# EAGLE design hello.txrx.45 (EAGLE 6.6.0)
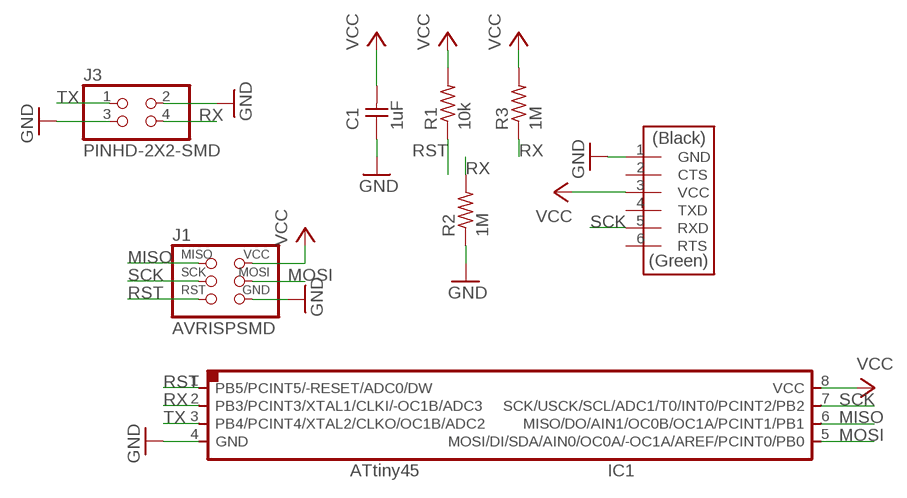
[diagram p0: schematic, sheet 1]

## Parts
C1  1uF  CAP-UNPOLARIZEDFAB  [C1206FAB]
IC1  ATTINY45SI  [SOIC8]
J1  AVRISPSMD  [2X03SMD]
J2  FTDI-SMD-HEADER  [1X06SMD]
J3  PINHD-2X2-SMD  [2X02SMD]
R1  10k  RES-US1206FAB  [R1206FAB]
R2  1M  RES-US1206FAB  [R1206FAB]
R3  1M  RES-US1206FAB  [R1206FAB]

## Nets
GND: C1.1 IC1.4(GND) J1.6(GND) J2.1(GND) J3.2 J3.3 R2.1
MISO: IC1.6(MISO/DO/AIN1/OC0B/OC1A/PCINT1/PB1) J1.1(MISO)
MOSI: IC1.5(MOSI/DI/SDA/AIN0/OC0A/-OC1A/AREF/PCINT0/PB0) J1.4(MOSI)
RST: IC1.1(PB5/PCINT5/-RESET/ADC0/DW) J1.5(RST) R1.1
RX: IC1.2(PB3/PCINT3/XTAL1/CLKI/-OC1B/ADC3) J3.4 R2.2 R3.1
SCK: IC1.7(SCK/USCK/SCL/ADC1/T0/INT0/PCINT2/PB2) J1.3(SCK) J2.5(RXD)
TX: IC1.3(PB4/PCINT4/XTAL2/CLKO/OC1B/ADC2) J3.1
VCC: C1.2 IC1.8(VCC) J1.2(VCC) J2.3(VCC) R1.2 R3.2
Unconnected: J2.2(CTS) J2.4(TXD) J2.6(RTS)

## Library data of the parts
C1 = fab:CAP-UNPOLARIZED
IC1 = fab:ATTINY45
J1 = fab:AVRISP
J2 = fab:FTDI-SMD-HEADER
J3 = fab:PINHD-2X2-SMD
R1-R3 = fab:RES-US: Resistor (US Symbol)

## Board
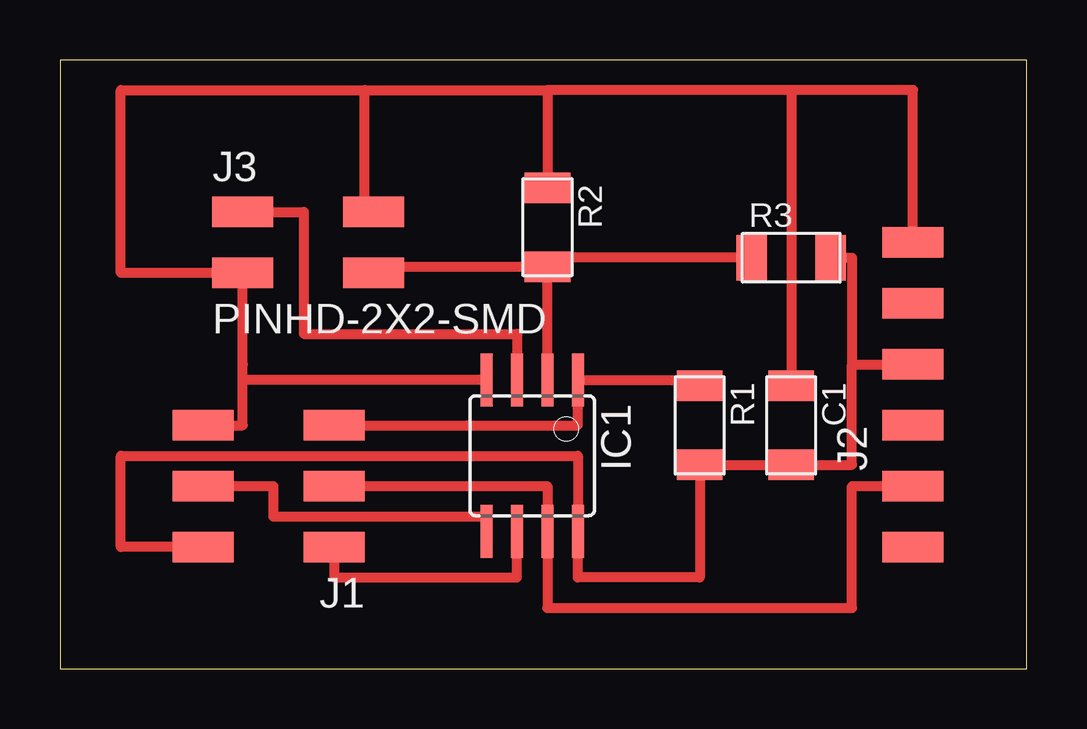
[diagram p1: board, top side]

Size 40.31 x 25.39 mm. Coordinates in mm from the lower left corner, seen from the top.
Outline: 0,0 40.31,0 40.31,25.39 0,25.39 0,0
Copper layers (1*16): Top 0.035mm / dielectric 1.5mm / Bottom 0.035mm
Design rules "fabmodule": minimum track width 10mil, minimum drill 0.4mm, track to track 0.42mm, track to pad 0.42mm, pad to pad 0.42mm, via to via 0.42mm, smd to smd 0.42mm, copper to edge 40mil, drill to drill 0.8mm, minimum pad ring 10mil, minimum via ring 8mil, stop-mask expansion 4mil, vias tented up to drill 0mil, thermal gap 10mil

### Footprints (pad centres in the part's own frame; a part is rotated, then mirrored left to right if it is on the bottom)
C1206FAB = smd 1.27 x 1.905: 1 -1.651,0; 2 1.651,0
SOIC8 = smd 0.5 x 2.2: 1 -1.905,-3.154; 2 -0.645,-3.154; 3 0.625,-3.154; 4 1.895,-3.154; 5 1.905,3.154; 6 0.635,3.154; 7 -0.635,3.154; 8 -1.905,3.154
2X03SMD = smd 2.54 x 1.27: 1 -2.54,2.54; 2 2.92,2.54; 3 -2.54,0; 4 2.92,0; 5 -2.54,-2.54; 6 2.92,-2.54
1X06SMD = smd 2.54 x 1.27: 1 0,6.35; 2 0,3.81; 3 0,1.27; 4 0,-1.27; 5 0,-3.81; 6 0,-6.35
2X02SMD = smd 2.54 x 1.27: 1 -2.54,1.27; 2 2.92,1.27; 3 -2.54,-1.27; 4 2.92,-1.27
R1206FAB = smd 1.27 x 1.905: 1 -1.651,0; 2 1.651,0

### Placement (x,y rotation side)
C1  30.48,10.16 270 top
IC1  19.69,8.89 180 top
J1  8.89,7.62 180 top
J2  35.56,11.43 0 top
J3  10.16,17.78 0 top
R1  26.67,10.16 270 top
R2  20.32,18.42 270 top
R3  30.48,17.14 0 top

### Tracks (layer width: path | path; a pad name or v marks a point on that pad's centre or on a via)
GND
  Top 0.406: J2.1 35.56,24.13 30.48,24.13 | 30.48,24.13 20.32,24.13 | 20.32,24.13 R2.1 | J3.2 12.7,19.05 12.7,24.13 | 12.7,24.13 20.32,24.13 | 12.7,24.13 2.54,24.13 2.54,16.51 J3.3 7.62,12.7 7.62,12.04 | 30.48,24.13 C1.1 | J1.6 7.62,10.16 7.62,12.04 | IC1.4 7.62,12.04
MISO
  Top 0.406: J1.1 11.43,3.81 19.05,3.81 IC1.6
MOSI
  Top 0.406: J1.4 8.89,7.62 8.89,6.35 17.78,6.35 IC1.5
RST
  Top 0.406: R1.1 26.67,12.04 IC1.1 21.59,10.16 J1.5
RX
  Top 0.406: R3.1 20.32,17.14 R2.2 | IC1.2 R2.2 | R2.2 13.08,16.76 J3.4
SCK
  Top 0.406: J1.3 20.32,7.62 IC1.7 20.32,2.54 33.02,2.54 33.02,7.62 J2.5
TX
  Top 0.406: J3.1 10.16,19.05 10.16,13.97 19.06,13.97 IC1.3
VCC
  Top 0.406: R3.2 33.02,17.14 33.02,12.7 | 33.02,12.7 J2.3 | 33.02,12.7 33.02,8.51 C1.2 R1.2 26.67,3.81 21.59,3.81 IC1.8 21.59,8.89 2.54,8.89 2.54,5.08 J1.2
